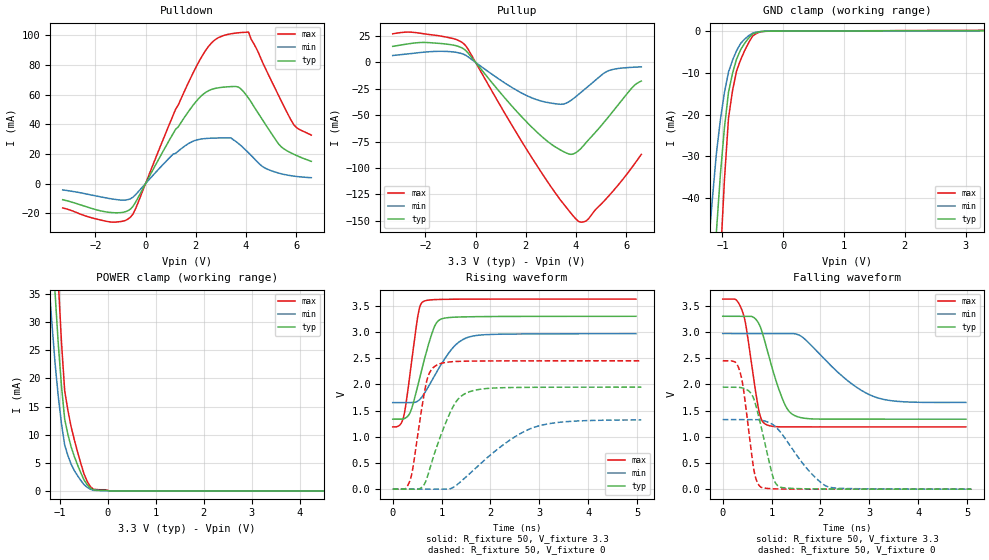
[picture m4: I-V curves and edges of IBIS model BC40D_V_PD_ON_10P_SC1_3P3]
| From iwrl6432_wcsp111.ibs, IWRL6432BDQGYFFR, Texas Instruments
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|   Model Cell BC40D_V_PD_ON_10P_SC1_3P3
|BC40D_V_PD_ON_10P_SC1_3P3
[Model]   BC40D_V_PD_ON_10P_SC1_3P3
Model_type   I/O
Polarity   Non-Inverting
Enable   Active-Low
Vinl =  0.8V
Vinh =  2V
Cref =  15pF
Rref =  100.0000M
Vref =  0V
Vmeas =  1.65
C_comp   2.059994p   1.912853p   2.135747p
|[Input load] weak_pd_on
|[Output drive] slow
|[supplytol] 10
|[temp] ind
[Model Spec]
Vinl   0.8V   0.8V   0.8V
Vinh   2V   2V   2V
[Temperature Range]   25   125   -40
[Voltage Range]   3.3   2.97   3.63
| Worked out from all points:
|   slope of the pulldown table from 0 to 0.495 V, typ, clamps not added: 31.8 ohm
|   slope of the pullup table from 0 to 0.495 V, typ, clamps not added: 33.8 ohm
|   GND clamp passes 1 mA (typ) near -0.52 V on its own axis
|   POWER clamp passes 1 mA (typ) near -0.42 V on its own axis
|   rising waveform, R_fixture 50, V_fixture 3.3: 20-80 % time 334ps typ, 532ps min, 208ps max; typ from 1.33 V to 3.3 V
|   rising waveform, R_fixture 50, V_fixture 0: 20-80 % time 466ps typ, 1.07ns min, 244ps max; typ from 0 V to 1.95 V
|   falling waveform, R_fixture 50, V_fixture 3.3: 20-80 % time 385ps typ, 931ps min, 233ps max; typ from 3.3 V to 1.33 V
|   falling waveform, R_fixture 50, V_fixture 0: 20-80 % time 293ps typ, 644ps min, 201ps max; typ from 1.95 V to 0 V
| Nom Voltages:
|   VDD=1.1001, VDDS=3.3, VDDS18=1.8, ESD_BIASFET=0, VSS=0, VSSS=0
| Min Voltages:
|   VDD=0.99, VDDS=2.97, VDDS18=1.62, ESD_BIASFET=0, VSS=0, VSSS=0
| Max Voltages:
|   VDD=1.21, VDDS=3.63, VDDS18=1.98, ESD_BIASFET=0, VSS=0, VSSS=0
[POWER_clamp]
|   voltage   I(typ)   I(min)   I(max)
-3.3V     446.9mA    419.5mA    603.9mA
-1.233V   56.59mA    37.53mA    80.37mA
-1.167V   45.68mA    29.91mA    65.17mA
-1.1V     35.14mA    22.67mA    50.36mA
-1.033V   26.13mA    16.78mA    37.31mA
-966.7mV  18.67mA    11.95mA    26.46mA
-900mV    12.76mA    8.172mA    17.82mA
-833.3mV  10.07mA    6.29mA     14.35mA
-566.7mV  3.276mA    1.904mA    4.983mA
-366.7mV  519.9uA    307.2uA    792.3uA
33.33mV   0A         0A         0A
6.6V      0A         0A         0A
[Pulldown]
|   voltage   I(typ)   I(min)   I(max)
-3.3V     -10.93mA   -4.311mA   -16.48mA
-1.4V     -19.53mA   -10.23mA   -25.96mA
-600mV    -17.23mA   -10.26mA   -22.66mA
1.1V      33.82mA    19.89mA    46.25mA
2V        55.14mA    29.24mA    78.29mA
2.6V      63.35mA    30.61mA    94.44mA
3.2V      65.21mA    30.81mA    100.4mA
3.7V      65.09mA    27.02mA    101.8mA
4.1V      57.64mA    20.71mA    102.2mA
5.3V      26.68mA    7.058mA    59.31mA
5.9V      19.77mA    5.007mA    39.76mA
6.6V      14.97mA    3.923mA    32.7mA
[Pullup]
|   voltage   I(typ)   I(min)   I(max)
-3.3V     15.12mA    6.498mA    27.02mA
-1.9V     18.73mA    9.943mA    26.53mA
-900mV    16.4mA     9.888mA    22.58mA
-400mV    11.39mA    6.786mA    15.98mA
2.4V      -65.08mA   -35.06mA   -96.18mA
3.5V      -84.52mA   -39.53mA   -134mA
3.8V      -87.17mA   -36.01mA   -143mA
4.1V      -83.69mA   -30.35mA   -150.6mA
4.4V      -75.99mA   -24.42mA   -150.3mA
5.3V      -51.41mA   -7.872mA   -126.6mA
6.3V      -22.29mA   -4.606mA   -97.15mA
6.6V      -17.71mA   -4.277mA   -87.2mA
[GND_clamp]
|   voltage   I(typ)   I(min)   I(max)
-3.3V     -787.2mA   -607.8mA   -1.235A
-1.233V   -85.66mA   -52.14mA   -138.8mA
-1.167V   -66.47mA   -40.37mA   -107.7mA
-1.1V     -48.25mA   -29.37mA   -77.99mA
-1.033V   -34.28mA   -21.19mA   -54.56mA
-966.7mV  -23.07mA   -14.67mA   -35.51mA
-900mV    -14.62mA   -9.792mA   -20.84mA
-833.3mV  -10.07mA   -6.938mA   -14.17mA
-700mV    -4.435mA   -2.939mA   -6.836mA
-500mV    -641.2uA   -454.5uA   -1.12mA
-300mV    -31.62uA   -32.73uA   -44.27uA
3.3V      108.6uA    159.4uA    198.5uA
[Ramp]
| variable   typ   min   max
dV/dt_f  1.1800539/0.38506764n 0.79469436/0.93858809n  1.4663953/0.23379182n
dV/dt_r  1.1731734/0.46682563n 0.80227934/1.080283n   1.4754285/0.24457461n
R_load = 50
[Rising Waveform]
R_fixture = 50
V_fixture = 3.3
V_fixture_min = 2.97
V_fixture_max = 3.63
|   time   V(typ)   V(min)   V(max)
0s        1.335V     1.651V     1.187V
223.4ps   1.341V     1.651V     1.381V
365.8ps   1.482V     1.651V     2.282V
518.6ps   1.998V     1.684V     3.33V
630.3ps   2.415V     1.802V     3.582V
810.3ps   2.992V     2.09V      3.614V
921.6ps   3.202V     2.274V     3.619V
1.262ns   3.281V     2.729V     3.624V
1.555ns   3.289V     2.902V     3.625V
4.974ns   3.298V     2.966V     3.627V
[Rising Waveform]
R_fixture = 50
V_fixture = 0
V_fixture_min = 0
V_fixture_max = 0
|   time   V(typ)   V(min)   V(max)
0s        0V         0V         0V
249.1ps   0V         0V         0V
353.3ps   0V         0V         165.9mV
568ps     16.56mV    0V         1.387V
691.3ps   186.6mV    0V         2.047V
902.7ps   815.8mV    0V         2.368V
1.276ns   1.642V     57.01mV    2.435V
1.614ns   1.872V     330.6mV    2.443V
2.938ns   1.944V     1.194V     2.449V
5.085ns   1.946V     1.321V     2.449V
[Falling Waveform]
R_fixture = 50
V_fixture = 3.3
V_fixture_min = 2.97
V_fixture_max = 3.63
|   time   V(typ)   V(min)   V(max)
0s        3.298V     2.969V     3.626V
269.8ps   3.298V     2.969V     3.614V
406.5ps   3.298V     2.969V     3.383V
483ps     3.298V     2.969V     3.075V
735.8ps   3.162V     2.969V     1.517V
887.5ps   2.728V     2.969V     1.233V
1.253ns   1.652V     2.969V     1.188V
1.512ns   1.388V     2.956V     1.187V
3.068ns   1.335V     1.774V     1.186V
4.974ns   1.334V     1.654V     1.186V
[Falling Waveform]
R_fixture = 50
V_fixture = 0
V_fixture_min = 0
V_fixture_max = 0
|   time   V(typ)   V(min)   V(max)
0s        1.945V     1.327V     2.448V
348.9ps   1.941V     1.327V     2.253V
428.9ps   1.924V     1.327V     1.879V
639.9ps   1.712V     1.327V     355.4mV
786.5ps   1.188V     1.317V     36.13mV
1.032ns   222.4mV    1.227V     6.608mV
1.187ns   36.69mV    1.082V     3.214mV
1.739ns   6.423mV    374.9mV    0V
2.167ns   3.049mV    42.27mV    0V
5.085ns   0V         0V         0V
